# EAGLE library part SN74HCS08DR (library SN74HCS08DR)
Logic Gates 4-ch, 2-input, 2-V to 6-V low power AND gates with Schmitt-Trigger inputs 14-SOIC -40 to 125 Source: Datasheet
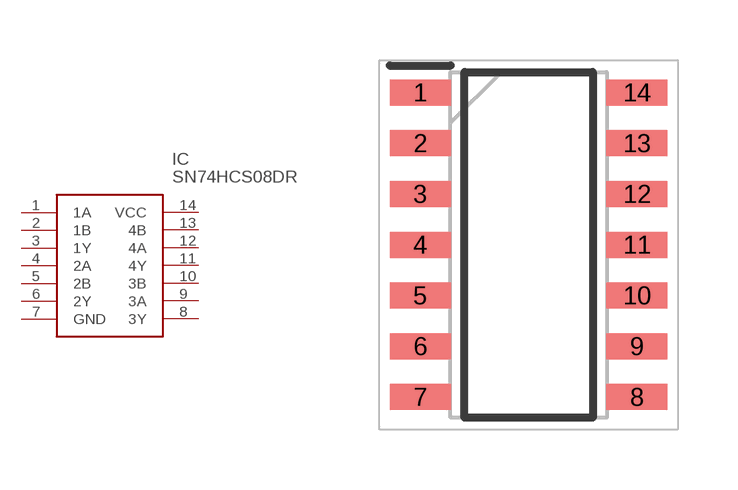
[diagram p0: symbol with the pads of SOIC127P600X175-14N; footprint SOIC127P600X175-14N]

Designator prefix IC

## SN74HCS08DR (Description: Logic Gates 4-ch, 2-input, 2-V to 6-V low power AND gates with Schmitt-Trigger inputs 14-SOIC -40 to 125; Height: 1.75mm; Manufacturer_Name: Texas Instruments; Manufacturer_Part_Number: SN74HCS08DR; Mouser_Part_Number: 595-SN74HCS08DR; Mouser_Price-Stock: https://www.mouser.co.uk/ProductDetail/Texas-Instruments/SN74HCS08DR?qs=7MVldsJ5UaxBpqBusi11%2Fg%3D%3D)  [SOIC127P600X175-14N]
1  1A
2  1B
3  1Y
4  2A
5  2B
6  2Y
7  GND
8  3Y
9  3A
10  3B
11  4Y
12  4A
13  4B
14  VCC

## Footprint SOIC127P600X175-14N (pad centres in mm)
D (-R-PDSO-G14)
smd 1.525 x 0.65: 1 -2.712,3.81; 2 -2.712,2.54; 3 -2.712,1.27; 4 -2.712,0; 5 -2.712,-1.27; 6 -2.712,-2.54; 7 -2.712,-3.81; 8 2.712,-3.81; 9 2.712,-2.54; 10 2.712,-1.27; 11 2.712,0; 12 2.712,1.27; 13 2.712,2.54; 14 2.712,3.81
